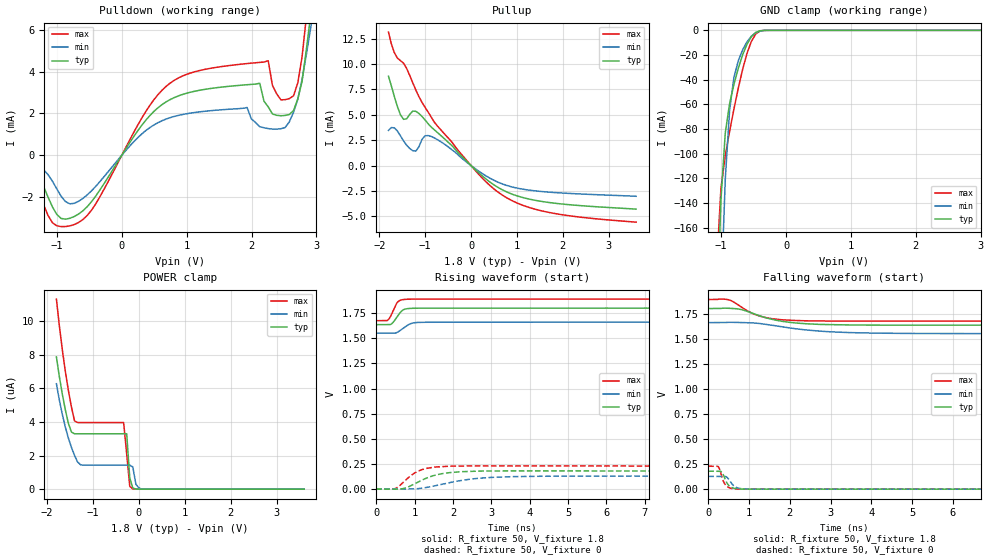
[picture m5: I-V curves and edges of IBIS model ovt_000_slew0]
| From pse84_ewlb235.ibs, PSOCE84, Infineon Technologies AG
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[Model] ovt_000_slew0
Model_type I/O
Enable   Active-High
Vinl  =  0.54
Vinh  =  1.26
Vmeas =  0.9
Cref  =  15e-12
| Capacitance   typ   min   max
C_comp   1.39974e-12   1.35992e-12   1.44753e-12
| Variables   typ   min   max
[GND Clamp Reference]   0   0   0
[POWER Clamp Reference]   1.8   1.66   1.89
[Pulldown Reference]   0   0   0
[Pullup Reference]   1.8   1.66   1.89
[Temperature Range]   25   125   -40
[Voltage Range]   1.8   1.66   1.89
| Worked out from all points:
|   slope of the pulldown table from 0 to 0.27 V, typ, clamps not added: 212 ohm
|   slope of the pullup table from 0 to 0.27 V, typ, clamps not added: 243 ohm
|   GND clamp passes 1 mA (typ) near -0.43 V on its own axis
|   falling waveform, R_fixture 50, V_fixture 1.8: 20-80 % time 893ps typ, 1.32ns min, 632ps max; typ from 1.8 V to 1.64 V
|   falling waveform, R_fixture 50, V_fixture 0: 20-80 % time 137ps typ, 156ps min, 126ps max; typ from 0.179 V to 0 V
|   rising waveform, R_fixture 50, V_fixture 1.8: 20-80 % time 191ps typ, 250ps min, 159ps max; typ from 1.64 V to 1.8 V
|   rising waveform, R_fixture 50, V_fixture 0: 20-80 % time 672ps typ, 1.09ns min, 475ps max; typ from 0 V to 0.179 V
[GND Clamp]
| Voltage   I(typ)   I(min)   I(max)
-1.271V   -717.5mA   -832.8mA   -643.6mA
-1.07V    -241.9mA   -348.3mA   -192.2mA
-1.003V   -137.2mA   -218.1mA   -128.1mA
-936.6mV  -83.06mA   -120.7mA   -101.3mA
-869.7mV  -59.26mA   -64.32mA   -81.77mA
-802.8mV  -43.7mA    -38.08mA   -63.69mA
-735.9mV  -30.76mA   -24.63mA   -46.83mA
-602.1mV  -11.27mA   -9.362mA   -18.72mA
-535.2mV  -5.241mA   -4.803mA   -9.042mA
-468.3mV  -1.746mA   -1.965mA   -3.086mA
-334.5mV  -35.9uA    -120.8uA   -33.39uA
3.6V      0A         0A         0A
[POWER Clamp]
| Voltage   I(typ)   I(min)   I(max)
-1.8V     7.872uA    6.273uA    11.31uA
-1.672V   5.671uA    4.461uA    8.32uA
-1.539V   3.91uA     3.037uA    5.87uA
-1.405V   3.295uA    2.008uA    4.063uA
-1.271V   3.295uA    1.447uA    3.964uA
-334.5mV  3.295uA    1.429uA    3.964uA
-267.6mV  3.295uA    1.429uA    2.099uA
-200.7mV  664.1nA    1.429uA    166.6nA
-133.8mV  69.92nA    1.319uA    14.86nA
-66.9mV   7.33nA     291.5nA    4.066nA
62.07mV   0A         0A         0A
3.6V      0A         0A         0A
[Pulldown]
| Voltage   I(typ)   I(min)   I(max)
-1.8V     -204uA     -190.9uA   -187.1uA
-1.405V   -550.3uA   -383.9uA   -779.9uA
-1.07V    -2.483mA   -1.25mA    -3.241mA
-735.9mV  -2.945mA   -2.313mA   -3.33mA
744.8mV   2.665mA    1.797mA    3.453mA
2.126V    3.446mA    1.362mA    4.446mA
2.256V    2.317mA    1.273mA    4.526mA
2.517V    1.903mA    1.322mA    2.66mA
2.712V    2.697mA    2.683mA    3.466mA
2.843V    5.026mA    4.793mA    6.577mA
2.908V    6.638mA    6.038mA    8.251mA
3.6V      22.12mA    6.161mA    25.65mA
[Pullup]
| Voltage   I(typ)   I(min)   I(max)
-1.8V     8.791mA    3.461mA    13.13mA
-1.672V   6.794mA    3.714mA    11.11mA
-1.472V   4.551mA    2.426mA    10.08mA
-1.271V   5.36mA     1.467mA    8.147mA
-1.137V   5.127mA    1.849mA    6.791mA
-1.003V   4.495mA    2.928mA    5.737mA
-869.7mV  3.801mA    2.866mA    4.778mA
124.1mV   -530.6uA   -410.2uA   -639.7uA
558.6mV   -2.068mA   -1.575mA   -2.506mA
993.1mV   -2.963mA   -2.204mA   -3.658mA
1.614V    -3.576mA   -2.58mA    -4.528mA
3.6V      -4.282mA   -3.02mA    -5.569mA
[Ramp]
dV/dt_r   0.107423/0.671771n  76.4267m/1.08695n  0.137218/0.475081n
dV/dt_f   98.8496m/0.893081n  65.342m/1.32407n  0.129087/0.632356n
R_load = 50
[Falling Waveform]
R_fixture = 50
V_fixture = 1.8
V_fixture_min = 1.66
V_fixture_max = 1.89
| Time   V(typ)   V(min)   V(max)
0s        1.8V       1.66V      1.89V
522.6ps   1.802V     1.663V     1.885V
763.9ps   1.794V     1.661V     1.828V
1.057ns   1.758V     1.658V     1.757V
1.276ns   1.726V     1.65V      1.723V
1.55ns    1.694V     1.635V     1.7V
2.354ns   1.649V     1.589V     1.678V
3.718ns   1.636V     1.558V     1.674V
6.615ns   1.635V     1.55V      1.675V
800ns     1.635V     1.551V     1.675V
[Falling Waveform]
R_fixture = 50
V_fixture = 0
V_fixture_min = 0
V_fixture_max = 0
| Time   V(typ)   V(min)   V(max)
0s        179mV      127.4mV    228.7mV
247.7ps   178.9mV    127.4mV    223.7mV
284.2ps   179.2mV    127.4mV    193.4mV
340.5ps   166.2mV    127.3mV    116.5mV
404.4ps   110.2mV    127.5mV    54.01mV
485.4ps   45.63mV    108.1mV    20.87mV
597.7ps   13.65mV    45.64mV    5.623mV
681.7ps   5.104mV    18.92mV    1.971mV
1.002ns   267.8uV    547.2uV    262.8uV
800ns     41.07nV    1.897uV    20.44nV
[Rising Waveform]
R_fixture = 50
V_fixture = 1.8
V_fixture_min = 1.66
V_fixture_max = 1.89
| Time   V(typ)   V(min)   V(max)
0s        1.635V     1.551V     1.675V
307.1ps   1.635V     1.551V     1.681V
404.3ps   1.644V     1.551V     1.74V
532.1ps   1.705V     1.556V     1.846V
577.2ps   1.73V      1.565V     1.866V
648.3ps   1.765V     1.584V     1.88V
766.6ps   1.791V     1.617V     1.888V
982.7ps   1.799V     1.654V     1.889V
1.662ns   1.8V       1.66V      1.89V
800ns     1.8V       1.66V      1.89V
[Rising Waveform]
R_fixture = 50
V_fixture = 0
V_fixture_min = 0
V_fixture_max = 0
| Time   V(typ)   V(min)   V(max)
0s        41.07nV    1.896uV    20.45nV
501ps     -1.107mV   -358.6uV   5.462mV
731.8ps   6.792mV    -750.9uV   75.66mV
961.7ps   43.35mV    503.5uV    149.7mV
1.333ns   111.6mV    16.96mV    207mV
1.711ns   152.5mV    47.24mV    223.1mV
2.411ns   174.8mV    96.06mV    230.3mV
3.548ns   180.5mV    123.2mV    229.7mV
5.771ns   179.6mV    128.5mV    228.8mV
800ns     179mV      127.4mV    228.7mV
